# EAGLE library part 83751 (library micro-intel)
MICROCOMPUTER/PERIPHERAL DEVICE
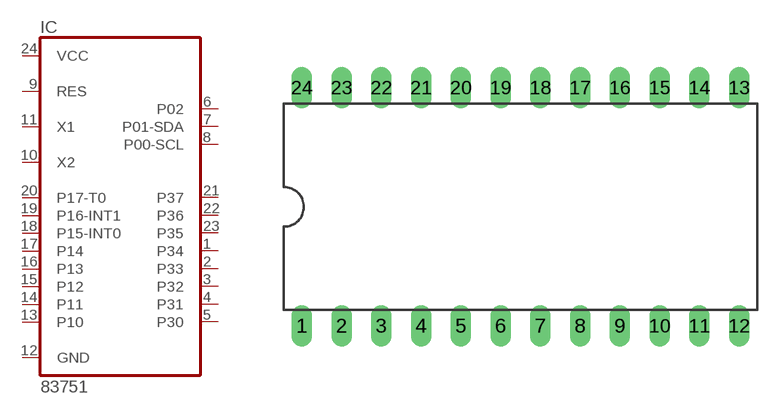
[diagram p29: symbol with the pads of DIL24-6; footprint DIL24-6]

Designator prefix IC

## 83751 (OC_FARNELL: unknown; OC_NEWARK: unknown)  [DIL24-6]
1  P34
2  P33
3  P32
4  P31
5  P30
6  P02
7  P01-SDA
8  P00-SCL
9  RES  in
10  X2  in
11  X1  in
12  GND  pwr
13  P10
14  P11
15  P12
16  P13
17  P14
18  P15-INT0
19  P16-INT1
20  P17-T0
21  P37
22  P36
23  P35
24  VCC  pwr

## Footprint DIL24-6 (pad centres in mm)
Dual In Line Package 0.6 inch
drill 0.813 long: 1 -13.97,-7.62; 2 -11.43,-7.62; 3 -8.89,-7.62; 4 -6.35,-7.62; 5 -3.81,-7.62; 6 -1.27,-7.62; 7 1.27,-7.62; 8 3.81,-7.62; 9 6.35,-7.62; 10 8.89,-7.62; 11 11.43,-7.62; 12 13.97,-7.62; 13 13.97,7.62; 14 11.43,7.62; 15 8.89,7.62; 16 6.35,7.62; 17 3.81,7.62; 18 1.27,7.62; 19 -1.27,7.62; 20 -3.81,7.62; 21 -6.35,7.62; 22 -8.89,7.62; 23 -11.43,7.62; 24 -13.97,7.62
